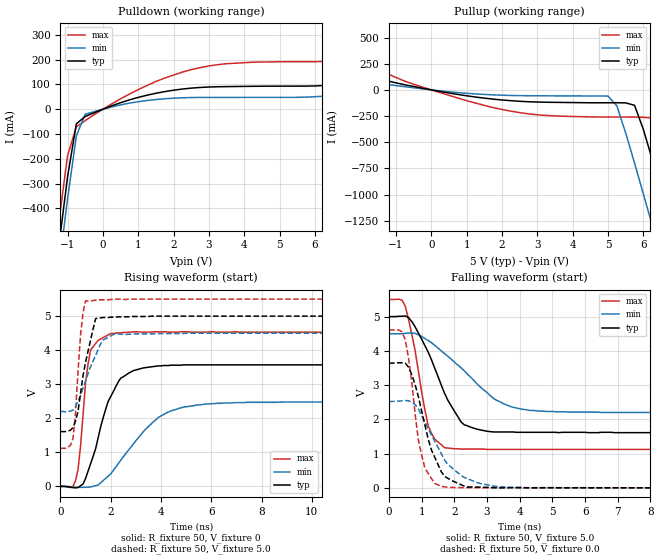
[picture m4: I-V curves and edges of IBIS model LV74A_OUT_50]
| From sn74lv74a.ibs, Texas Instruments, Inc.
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|   Model LV74A_OUT_50
[Model]   LV74A_OUT_50
Model_type  Output
Polarity   Non-Inverting
Vmeas = 2.50v
Cref = 15pf
| variable   typ   min   max
C_comp   4.62pf   3.47pf   5.77pf
[Temperature Range]   25   85   -40
[Voltage Range]   5.0   4.5   5.5
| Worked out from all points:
|   slope of the pulldown table from 0 to 0.75 V, typ, clamps not added: 19.9 ohm
|   slope of the pullup table from 0 to 0.75 V, typ, clamps not added: 17.2 ohm
|   rising waveform, R_fixture 50, V_fixture 0: 20-80 % time 929ps typ, 1.71ns min, 347ps max; typ from 0 V to 3.57 V
|   falling waveform, R_fixture 50, V_fixture 5.0: 20-80 % time 961ps typ, 1.59ns min, 495ps max; typ from 5 V to 1.61 V
|   rising waveform, R_fixture 50, V_fixture 5.0: 20-80 % time 492ps typ, 718ps min, 248ps max; typ from 1.61 V to 5 V
|   falling waveform, R_fixture 50, V_fixture 0.0: 20-80 % time 650ps typ, 976ps min, 395ps max; typ from 3.64 V to 0 V
[Pulldown]
|   Voltage   I(typ)   I(min)   I(max)
-5V       -5.14A     -5.22A     -5.05A
-1.5V     -853mA     -945mA     -756mA
-1.25V    -557mA     -649mA     -461mA
-1V       -274mA     -363mA     -188mA
-750mV    -58.9mA    -108mA     -71.3mA
-500mV    -29.2mA    -20mA      -46.2mA
0V        -3.33nA    -3.4nA     -3.57nA
1.25V     56.7mA     35.2mA     96mA
2.5V      85.3mA     47.3mA     160mA
3.5V      91.4mA     47.8mA     184mA
6.75V     103mA      58.5mA     199mA
10V       179mA      107mA      329mA
[Pullup]
|   Voltage   I(typ)   I(min)   I(max)
-5V       310mA      167mA      586mA
-3.5V     252mA      143mA      464mA
-750mV    48.6mA     30.8mA     83.5mA
1.5V      -78.8mA    -43.4mA    -148mA
5V        -123mA     -58.9mA    -259mA
5.25V     -123mA     -153mA     -259mA
5.75V     -147mA     -699mA     -260mA
6.25V     -664mA     -1.29A     -268mA
6.5V      -960mA     -1.6A      -403mA
6.75V     -1.26A     -1.9A      -685mA
7.25V     -1.87A     -2.51A     -1.28A
10V       -5.25A     -5.89A     -4.66A
[Ramp]
| variable   typ   min   max
dV/dt_r   2.15E+00/8.31E-10   1.50E+00/1.74E-09   2.72E+00/3.29E-10
dV/dt_f   2.05E+00/9.30E-10   1.39E+00/1.60E-09   2.64E+00/5.40E-10
R_load = 50
[Rising Waveform]
R_fixture = 50
V_fixture = 0
|   Time   V(typ)   V(min)   V(max)
0s        0V         0V         0V
600ps     -42.5mV    -24.2mV    167mV
800ps     19.8mV     -28.7mV    1.19V
1ns       236mV      -25.9mV    3.05V
1.2ns     668mV      -14.9mV    4.01V
2ns       2.64V      368mV      4.49V
2.4ns     3.18V      770mV      4.51V
3.9ns     3.54V      2.03V      4.54V
5.4ns     3.57V      2.39V      4.53V
25ns      3.57V      2.48V      4.53V
[Falling Waveform]
R_fixture = 50
V_fixture = 5.0
V_fixture_min = 4.5
V_fixture_max = 5.5
|   Time   V(typ)   V(min)   V(max)
0s        5V         4.5V       5.5V
400ps     5.01V      4.5V       5.48V
500ps     5.02V      4.51V      5.3V
800ps     4.7V       4.51V      4V
1.2ns     3.96V      4.3V       1.81V
1.7ns     2.76V      3.92V      1.17V
2.3ns     1.84V      3.42V      1.13V
3.3ns     1.63V      2.55V      1.12V
4.3ns     1.62V      2.26V      1.12V
25ns      1.61V      2.2V       1.12V
[Rising Waveform]
R_fixture = 50
V_fixture = 5.0
V_fixture_min = 4.5
V_fixture_max = 5.5
|   Time   V(typ)   V(min)   V(max)
0s        1.61V      2.2V       1.12V
500ps     1.73V      2.24V      1.41V
600ps     1.92V      2.34V      2.16V
800ps     2.74V      2.67V      4.45V
900ps     3.26V      2.89V      5.11V
1ns       3.65V      3.1V       5.45V
1.4ns     4.93V      3.85V      5.47V
1.7ns     4.96V      4.3V       5.48V
2.2ns     4.97V      4.48V      5.5V
25ns      5V         4.5V       5.5V
[Falling Waveform]
R_fixture = 50
V_fixture = 0.0
|   Time   V(typ)   V(min)   V(max)
0s        3.64V      2.52V      4.61V
500ps     3.64V      2.55V      4.32V
700ps     3.3V       2.5V       3.06V
900ps     2.66V      2.3V       1.39V
1ns       2.24V      2.11V      951mV
1.3ns     1.1V       1.54V      270mV
1.6ns     470mV      998mV      40.2mV
2.3ns     49.4mV     305mV      3.71mV
3.7ns     3.74mV     14.2mV     1.32mV
25ns      8.94uV     2.49uV     9.76uV
